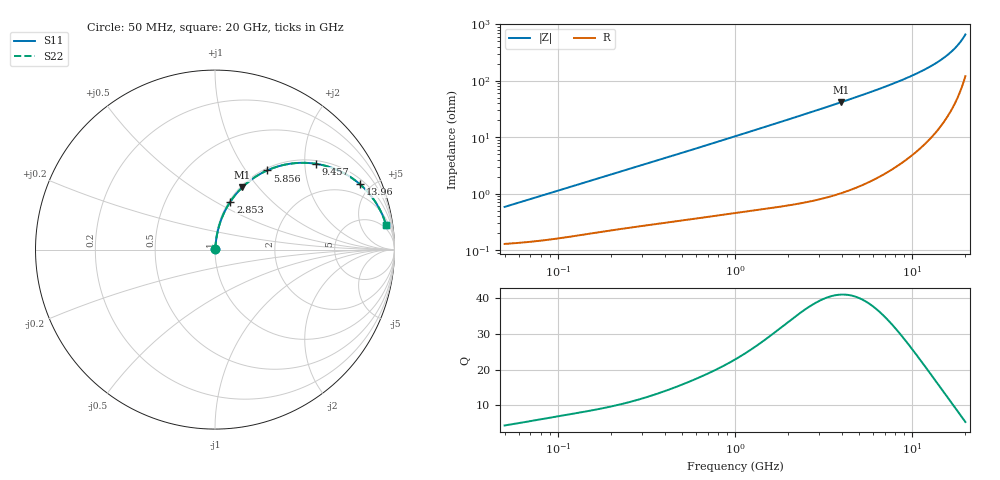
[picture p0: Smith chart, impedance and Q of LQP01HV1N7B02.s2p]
!Murata Part Number: LQP01HV1N7B02
!These Parameters are Measured in Series Mode Connection
!  o--[Z]--o
!Port1  Port2
!  o-------o
!Freq. Start=50[MHz] Stop=20[GHz], 401[Steps]
# Hz S RI R 50
!Freq.(Hz) S11(Real) S11(Imag) S21(Real) S21(Imag) S12(Real) S12(Imag) S22(Real) S22(Imag)
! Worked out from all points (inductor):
!   401 points, 50 MHz to 20 GHz, reference 50 ohm
!   read as one part in series: L = 1.8 nH near 51.52 MHz
!   highest Q = 40.9 at 3.967 GHz (marker M1), where L = 1.66 nH
!   S11 on the Smith chart (normalised r, x): 50 MHz: 1.00, +0.01; 2.853 GHz: 1.02, +0.59; 5.856 GHz: 1.03, +1.27; 9.457 GHz: 1.08, +2.27; 13.96 GHz: 1.27, +4.28; 20 GHz: 3, +13
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5e7  0.00132 0.00566  0.9987 -0.00566  0.9987 -0.00566  0.00132 0.00566
1.364002e8  0.00208 0.015  0.9979 -0.015  0.9979 -0.015  0.00208 0.015
3.721004e8  0.00446 0.0391  0.9955 -0.0391  0.9955 -0.0391  0.00446 0.0391
6.285508e8  0.0079 0.0648  0.9921 -0.0648  0.9921 -0.0648  0.0079 0.0648
1e9  0.0149 0.1013  0.9851 -0.1013  0.9851 -0.1013  0.0149 0.1013
1.689197e9  0.0344 0.1667  0.9656 -0.1667  0.9656 -0.1667  0.0344 0.1667
2.728004e9  0.0792 0.2573  0.9208 -0.2573  0.9208 -0.2573  0.0792 0.2573
2.853386e9  0.0858 0.2674  0.9142 -0.2674  0.9142 -0.2674  0.0858 0.2674
3.967106e9  0.1528 0.3478  0.8472 -0.3478  0.8472 -0.3478  0.1528 0.3478
4.81993e9  0.2126 0.3969  0.7874 -0.3969  0.7874 -0.3969  0.2126 0.3969
5.856089e9  0.2909 0.4412  0.7091 -0.4412  0.7091 -0.4412  0.2909 0.4412
7.442007e9  0.4143 0.4778  0.5857 -0.4778  0.5857 -0.4778  0.4143 0.4778
8.389408e9  0.4858 0.4836  0.5142 -0.4836  0.5142 -0.4836  0.4858 0.4836
9.457416e9  0.5618 0.4782  0.4382 -0.4782  0.4382 -0.4782  0.5618 0.4782
1.149051e10  0.6884 0.4407  0.3116 -0.4407  0.3116 -0.4407  0.6884 0.4407
1.276073e10  0.754 0.4047  0.246 -0.4047  0.246 -0.4047  0.754 0.4047
1.396067e10  0.8065 0.365  0.1935 -0.365  0.1935 -0.365  0.8065 0.365
1.550395e10  0.8613 0.3091  0.1387 -0.3091  0.1387 -0.3091  0.8613 0.3091
1.696185e10  0.9011 0.2537  0.0989 -0.2537  0.0989 -0.2537  0.9011 0.2537
1.828096e10  0.9283 0.2032  0.0717 -0.2032  0.0717 -0.2032  0.9283 0.2032
1.940974e10  0.9458 0.1604  0.0542 -0.1604  0.0542 -0.1604  0.9458 0.1604
2e10  0.953 0.1384  0.047 -0.1384  0.047 -0.1384  0.953 0.1384
